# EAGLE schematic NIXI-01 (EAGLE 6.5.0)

## Sheet 1 of 5: Anzeige 1+2
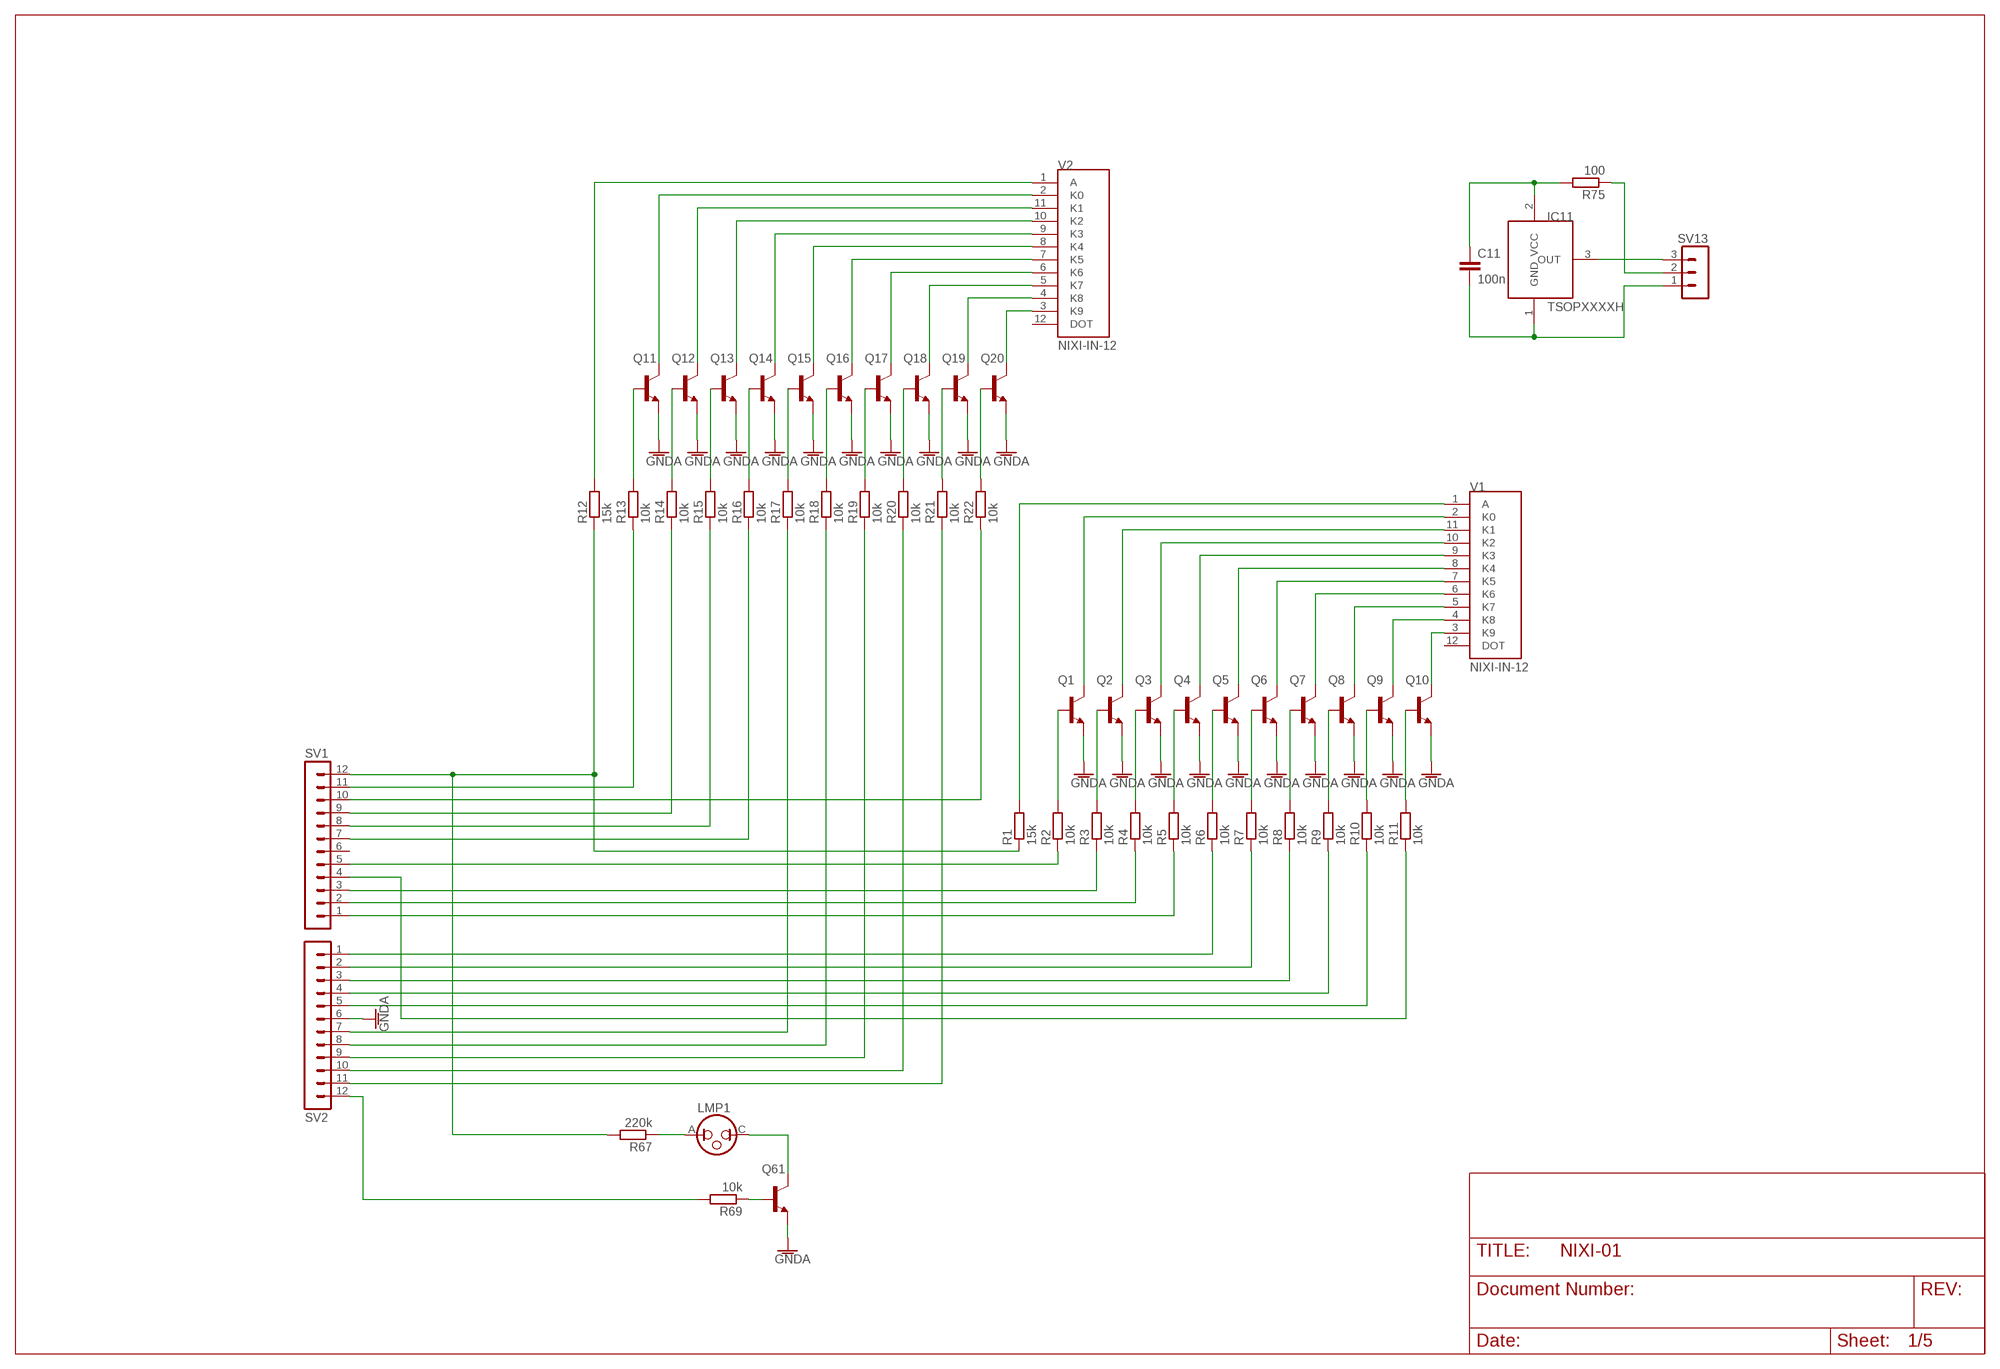
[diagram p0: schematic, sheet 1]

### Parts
C11  100n  C-EUC0603  [C0603]
IC11  TSOPXXXXH  [TSOPXXXX_H]
LMP1  NEON1  [NEONLAMP_6X28]
Q1  BC846ALT1SMD  [SOT23]
Q2  BC846ALT1SMD  [SOT23]
Q3  BC846ALT1SMD  [SOT23]
Q4  BC846ALT1SMD  [SOT23]
Q5  BC846ALT1SMD  [SOT23]
Q6  BC846ALT1SMD  [SOT23]
Q7  BC846ALT1SMD  [SOT23]
Q8  BC846ALT1SMD  [SOT23]
Q9  BC846ALT1SMD  [SOT23]
Q10  BC846ALT1SMD  [SOT23]
Q11  BC846ALT1SMD  [SOT23]
Q12  BC846ALT1SMD  [SOT23]
Q13  BC846ALT1SMD  [SOT23]
Q14  BC846ALT1SMD  [SOT23]
Q15  BC846ALT1SMD  [SOT23]
Q16  BC846ALT1SMD  [SOT23]
Q17  BC846ALT1SMD  [SOT23]
Q18  BC846ALT1SMD  [SOT23]
Q19  BC846ALT1SMD  [SOT23]
Q20  BC846ALT1SMD  [SOT23]
Q61  BC846ALT1SMD  [SOT23]
R1  15k  R-EU_R1206  [R1206]
R2  10k  R-EU_R0603  [R0603]
R3  10k  R-EU_R0603  [R0603]
R4  10k  R-EU_R0603  [R0603]
R5  10k  R-EU_R0603  [R0603]
R6  10k  R-EU_R0603  [R0603]
R7  10k  R-EU_R0603  [R0603]
R8  10k  R-EU_R0603  [R0603]
R9  10k  R-EU_R0603  [R0603]
R10  10k  R-EU_R0603  [R0603]
R11  10k  R-EU_R0603  [R0603]
R12  15k  R-EU_R1206  [R1206]
R13  10k  R-EU_R0603  [R0603]
R14  10k  R-EU_R0603  [R0603]
R15  10k  R-EU_R0603  [R0603]
R16  10k  R-EU_R0603  [R0603]
R17  10k  R-EU_R0603  [R0603]
R18  10k  R-EU_R0603  [R0603]
R19  10k  R-EU_R0603  [R0603]
R20  10k  R-EU_R0603  [R0603]
R21  10k  R-EU_R0603  [R0603]
R22  10k  R-EU_R0603  [R0603]
R67  220k  R-EU_R1206  [R1206]
R69  10k  R-EU_R0603  [R0603]
R75  100  R-EU_R0603  [R0603]
SV1  MA12-1  [MA12-1]
SV2  MA12-1  [MA12-1]
SV13  MA03-1  [MA03-1]
V1  NIXI-IN-12  [NIXI_IN-12]
V2  NIXI-IN-12  [NIXI_IN-12]

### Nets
GNDA: Q1.2(E) Q2.2(E) Q3.2(E) Q4.2(E) Q5.2(E) Q6.2(E) Q7.2(E) Q8.2(E) Q9.2(E) Q10.2(E) Q11.2(E) Q12.2(E) Q13.2(E) Q14.2(E) Q15.2(E) Q16.2(E) Q17.2(E) Q18.2(E) Q19.2(E) Q20.2(E) Q61.2(E) SV2.6 ; also sheet 2,3
N$1: R1.2 V1.1(A)
N$2: Q1.3(C) V1.2(K0)
N$3: Q2.3(C) V1.11(K1)
N$4: Q3.3(C) V1.10(K2)
N$5: Q4.3(C) V1.9(K3)
N$6: Q5.3(C) V1.8(K4)
N$7: Q6.3(C) V1.7(K5)
N$8: Q7.3(C) V1.6(K6)
N$9: Q8.3(C) V1.5(K7)
N$10: Q9.3(C) V1.4(K8)
N$11: Q10.3(C) V1.3(K9)
N$12: Q2.1(B) R3.2
N$13: Q3.1(B) R4.2
N$14: Q4.1(B) R5.2
N$15: Q5.1(B) R6.2
N$16: Q6.1(B) R7.2
N$17: Q7.1(B) R8.2
N$18: Q8.1(B) R9.2
N$19: Q9.1(B) R10.2
N$20: Q10.1(B) R11.2
N$21: Q1.1(B) R2.2
N$22: R5.1 SV1.1
N$23: R4.1 SV1.2
N$24: R3.1 SV1.3
N$25: R11.1 SV1.4
N$26: R2.1 SV1.5
N$28: R6.1 SV2.1
N$29: R7.1 SV2.2
N$30: R8.1 SV2.3
N$31: R9.1 SV2.4
N$32: R10.1 SV2.5
N$33: R12.2 V2.1(A)
N$34: Q11.3(C) V2.2(K0)
N$35: Q12.3(C) V2.11(K1)
N$36: Q13.3(C) V2.10(K2)
N$37: Q14.3(C) V2.9(K3)
N$38: Q15.3(C) V2.8(K4)
N$39: Q16.3(C) V2.7(K5)
N$40: Q17.3(C) V2.6(K6)
N$41: Q18.3(C) V2.5(K7)
N$42: Q19.3(C) V2.4(K8)
N$43: Q20.3(C) V2.3(K9)
N$44: Q12.1(B) R14.2
N$45: Q13.1(B) R15.2
N$46: Q14.1(B) R16.2
N$47: Q15.1(B) R17.2
N$48: Q16.1(B) R18.2
N$49: Q17.1(B) R19.2
N$50: Q18.1(B) R20.2
N$51: Q19.1(B) R21.2
N$52: Q20.1(B) R22.2
N$53: Q11.1(B) R13.2
N$54: R16.1 SV1.7
N$55: R15.1 SV1.8
N$56: R14.1 SV1.9
N$57: R22.1 SV1.10
N$58: R13.1 SV1.11
N$59: R1.1 R12.1 R67.2 SV1.12
N$60: R17.1 SV2.7
N$61: R18.1 SV2.8
N$62: R19.1 SV2.9
N$63: R20.1 SV2.10
N$64: R21.1 SV2.11
N$194: LMP1.C Q61.3(C)
N$195: LMP1.A R67.1
N$196: Q61.1(B) R69.1
N$197: R69.2 SV2.12
N$202: C11.2 IC11.1(GND) SV13.1
N$226: C11.1 IC11.2(VCC) R75.2
N$227: IC11.3(OUT) SV13.3
N$252: R75.1 SV13.2
Unconnected: SV1.6 V1.12(DOT) V2.12(DOT)

## Sheet 2 of 5: Anzeige 3+4
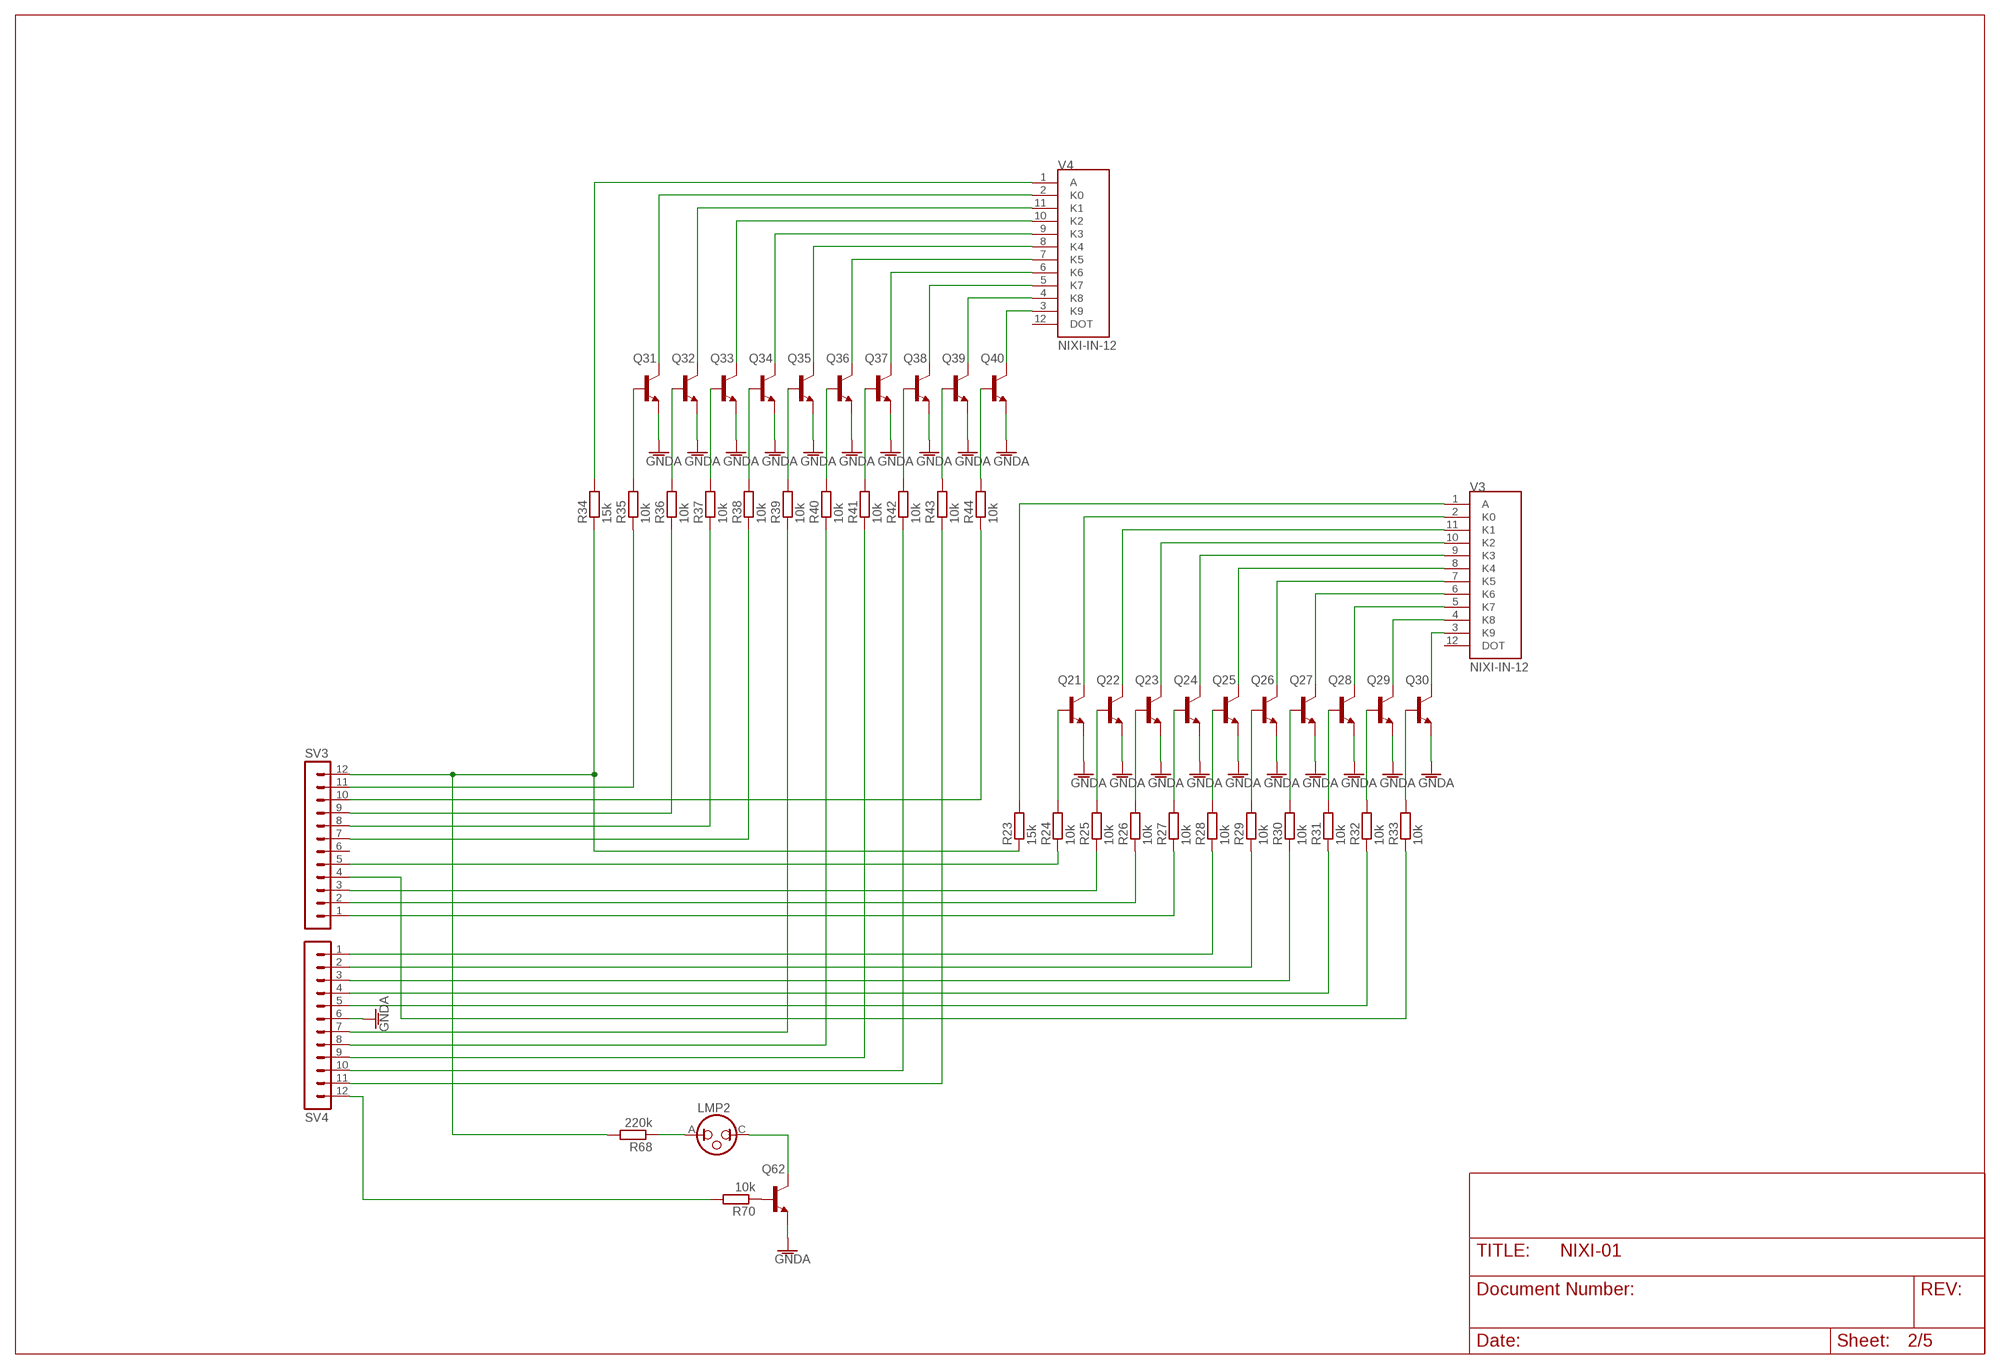
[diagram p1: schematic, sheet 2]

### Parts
LMP2  NEON1  [NEONLAMP_6X28]
Q21  BC846ALT1SMD  [SOT23]
Q22  BC846ALT1SMD  [SOT23]
Q23  BC846ALT1SMD  [SOT23]
Q24  BC846ALT1SMD  [SOT23]
Q25  BC846ALT1SMD  [SOT23]
Q26  BC846ALT1SMD  [SOT23]
Q27  BC846ALT1SMD  [SOT23]
Q28  BC846ALT1SMD  [SOT23]
Q29  BC846ALT1SMD  [SOT23]
Q30  BC846ALT1SMD  [SOT23]
Q31  BC846ALT1SMD  [SOT23]
Q32  BC846ALT1SMD  [SOT23]
Q33  BC846ALT1SMD  [SOT23]
Q34  BC846ALT1SMD  [SOT23]
Q35  BC846ALT1SMD  [SOT23]
Q36  BC846ALT1SMD  [SOT23]
Q37  BC846ALT1SMD  [SOT23]
Q38  BC846ALT1SMD  [SOT23]
Q39  BC846ALT1SMD  [SOT23]
Q40  BC846ALT1SMD  [SOT23]
Q62  BC846ALT1SMD  [SOT23]
R23  15k  R-EU_R1206  [R1206]
R24  10k  R-EU_R0603  [R0603]
R25  10k  R-EU_R0603  [R0603]
R26  10k  R-EU_R0603  [R0603]
R27  10k  R-EU_R0603  [R0603]
R28  10k  R-EU_R0603  [R0603]
R29  10k  R-EU_R0603  [R0603]
R30  10k  R-EU_R0603  [R0603]
R31  10k  R-EU_R0603  [R0603]
R32  10k  R-EU_R0603  [R0603]
R33  10k  R-EU_R0603  [R0603]
R34  15k  R-EU_R1206  [R1206]
R35  10k  R-EU_R0603  [R0603]
R36  10k  R-EU_R0603  [R0603]
R37  10k  R-EU_R0603  [R0603]
R38  10k  R-EU_R0603  [R0603]
R39  10k  R-EU_R0603  [R0603]
R40  10k  R-EU_R0603  [R0603]
R41  10k  R-EU_R0603  [R0603]
R42  10k  R-EU_R0603  [R0603]
R43  10k  R-EU_R0603  [R0603]
R44  10k  R-EU_R0603  [R0603]
R68  220k  R-EU_R1206  [R1206]
R70  10k  R-EU_R0603  [R0603]
SV3  MA12-1  [MA12-1]
SV4  MA12-1  [MA12-1]
V3  NIXI-IN-12  [NIXI_IN-12]
V4  NIXI-IN-12  [NIXI_IN-12]

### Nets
GNDA: Q21.2(E) Q22.2(E) Q23.2(E) Q24.2(E) Q25.2(E) Q26.2(E) Q27.2(E) Q28.2(E) Q29.2(E) Q30.2(E) Q31.2(E) Q32.2(E) Q33.2(E) Q34.2(E) Q35.2(E) Q36.2(E) Q37.2(E) Q38.2(E) Q39.2(E) Q40.2(E) Q62.2(E) SV4.6 ; also sheet 1,3
N$65: R23.2 V3.1(A)
N$66: Q21.3(C) V3.2(K0)
N$67: Q22.3(C) V3.11(K1)
N$68: Q23.3(C) V3.10(K2)
N$69: Q24.3(C) V3.9(K3)
N$70: Q25.3(C) V3.8(K4)
N$71: Q26.3(C) V3.7(K5)
N$72: Q27.3(C) V3.6(K6)
N$73: Q28.3(C) V3.5(K7)
N$74: Q29.3(C) V3.4(K8)
N$75: Q30.3(C) V3.3(K9)
N$76: Q22.1(B) R25.2
N$77: Q23.1(B) R26.2
N$78: Q24.1(B) R27.2
N$79: Q25.1(B) R28.2
N$80: Q26.1(B) R29.2
N$81: Q27.1(B) R30.2
N$82: Q28.1(B) R31.2
N$83: Q29.1(B) R32.2
N$84: Q30.1(B) R33.2
N$85: Q21.1(B) R24.2
N$86: R27.1 SV3.1
N$87: R26.1 SV3.2
N$88: R25.1 SV3.3
N$89: R33.1 SV3.4
N$90: R24.1 SV3.5
N$92: R28.1 SV4.1
N$93: R29.1 SV4.2
N$94: R30.1 SV4.3
N$95: R31.1 SV4.4
N$96: R32.1 SV4.5
N$97: R34.2 V4.1(A)
N$98: Q31.3(C) V4.2(K0)
N$99: Q32.3(C) V4.11(K1)
N$100: Q33.3(C) V4.10(K2)
N$101: Q34.3(C) V4.9(K3)
N$102: Q35.3(C) V4.8(K4)
N$103: Q36.3(C) V4.7(K5)
N$104: Q37.3(C) V4.6(K6)
N$105: Q38.3(C) V4.5(K7)
N$106: Q39.3(C) V4.4(K8)
N$107: Q40.3(C) V4.3(K9)
N$108: Q32.1(B) R36.2
N$109: Q33.1(B) R37.2
N$110: Q34.1(B) R38.2
N$111: Q35.1(B) R39.2
N$112: Q36.1(B) R40.2
N$113: Q37.1(B) R41.2
N$114: Q38.1(B) R42.2
N$115: Q39.1(B) R43.2
N$116: Q40.1(B) R44.2
N$117: Q31.1(B) R35.2
N$118: R38.1 SV3.7
N$119: R37.1 SV3.8
N$120: R36.1 SV3.9
N$121: R44.1 SV3.10
N$122: R35.1 SV3.11
N$124: R39.1 SV4.7
N$125: R40.1 SV4.8
N$126: R41.1 SV4.9
N$127: R42.1 SV4.10
N$128: R43.1 SV4.11
N$193: R23.1 R34.1 R68.2 SV3.12
N$198: LMP2.A R68.1
N$199: LMP2.C Q62.3(C)
N$200: Q62.1(B) R70.1
N$201: R70.2 SV4.12
Unconnected: SV3.6 V3.12(DOT) V4.12(DOT)

## Sheet 3 of 5: Anzeige 5+6
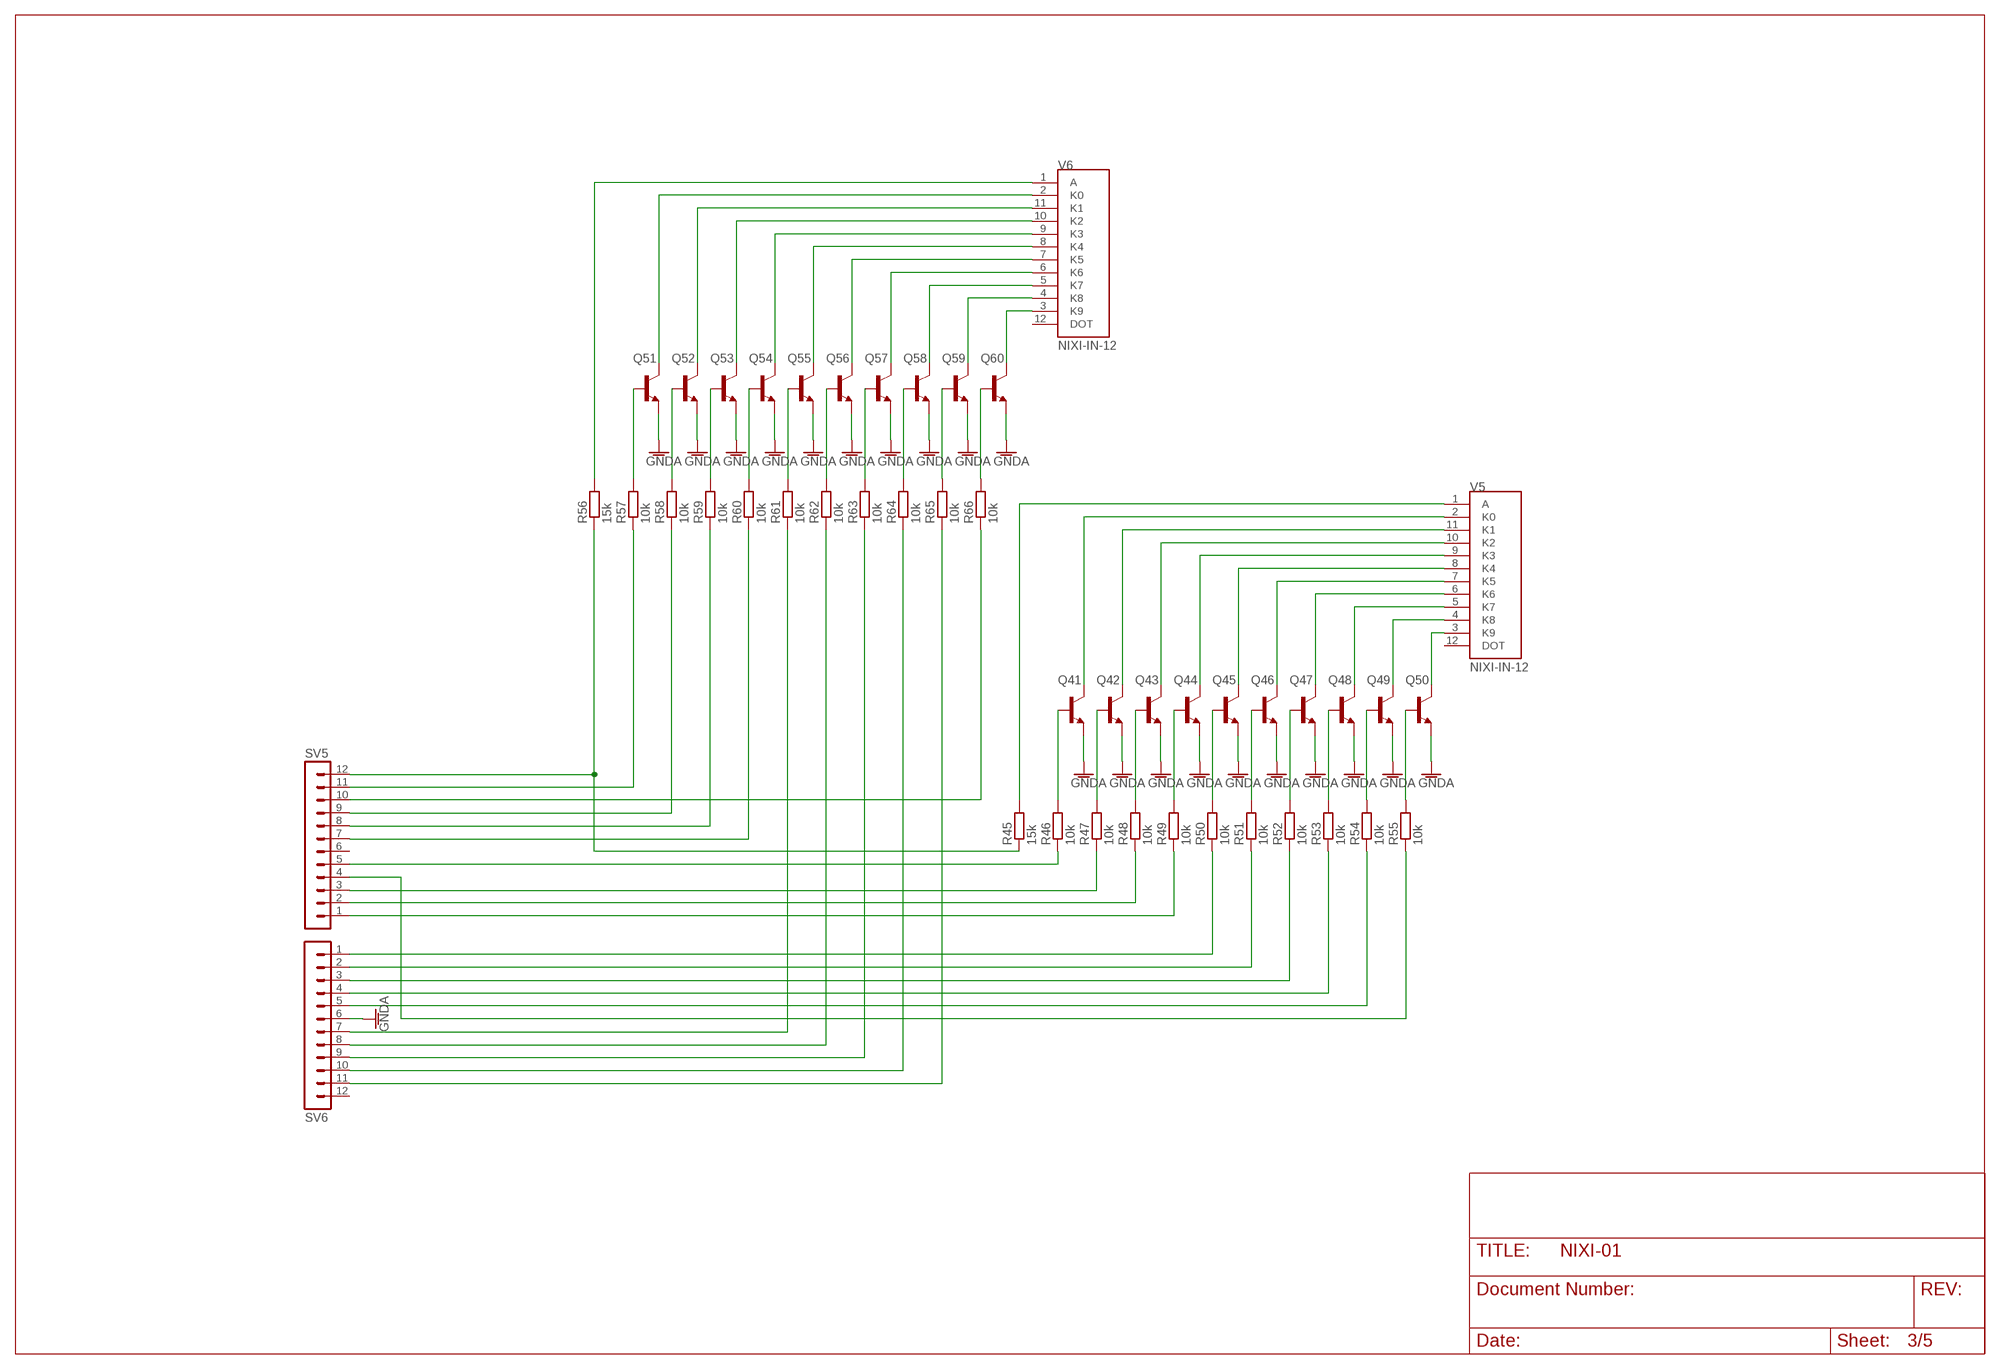
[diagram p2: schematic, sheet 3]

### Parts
Q41  BC846ALT1SMD  [SOT23]
Q42  BC846ALT1SMD  [SOT23]
Q43  BC846ALT1SMD  [SOT23]
Q44  BC846ALT1SMD  [SOT23]
Q45  BC846ALT1SMD  [SOT23]
Q46  BC846ALT1SMD  [SOT23]
Q47  BC846ALT1SMD  [SOT23]
Q48  BC846ALT1SMD  [SOT23]
Q49  BC846ALT1SMD  [SOT23]
Q50  BC846ALT1SMD  [SOT23]
Q51  BC846ALT1SMD  [SOT23]
Q52  BC846ALT1SMD  [SOT23]
Q53  BC846ALT1SMD  [SOT23]
Q54  BC846ALT1SMD  [SOT23]
Q55  BC846ALT1SMD  [SOT23]
Q56  BC846ALT1SMD  [SOT23]
Q57  BC846ALT1SMD  [SOT23]
Q58  BC846ALT1SMD  [SOT23]
Q59  BC846ALT1SMD  [SOT23]
Q60  BC846ALT1SMD  [SOT23]
R45  15k  R-EU_R1206  [R1206]
R46  10k  R-EU_R0603  [R0603]
R47  10k  R-EU_R0603  [R0603]
R48  10k  R-EU_R0603  [R0603]
R49  10k  R-EU_R0603  [R0603]
R50  10k  R-EU_R0603  [R0603]
R51  10k  R-EU_R0603  [R0603]
R52  10k  R-EU_R0603  [R0603]
R53  10k  R-EU_R0603  [R0603]
R54  10k  R-EU_R0603  [R0603]
R55  10k  R-EU_R0603  [R0603]
R56  15k  R-EU_R1206  [R1206]
R57  10k  R-EU_R0603  [R0603]
R58  10k  R-EU_R0603  [R0603]
R59  10k  R-EU_R0603  [R0603]
R60  10k  R-EU_R0603  [R0603]
R61  10k  R-EU_R0603  [R0603]
R62  10k  R-EU_R0603  [R0603]
R63  10k  R-EU_R0603  [R0603]
R64  10k  R-EU_R0603  [R0603]
R65  10k  R-EU_R0603  [R0603]
R66  10k  R-EU_R0603  [R0603]
SV5  MA12-1  [MA12-1]
SV6  MA12-1  [MA12-1]
V5  NIXI-IN-12  [NIXI_IN-12]
V6  NIXI-IN-12  [NIXI_IN-12]

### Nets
GNDA: Q41.2(E) Q42.2(E) Q43.2(E) Q44.2(E) Q45.2(E) Q46.2(E) Q47.2(E) Q48.2(E) Q49.2(E) Q50.2(E) Q51.2(E) Q52.2(E) Q53.2(E) Q54.2(E) Q55.2(E) Q56.2(E) Q57.2(E) Q58.2(E) Q59.2(E) Q60.2(E) SV6.6 ; also sheet 1,2
N$129: R45.2 V5.1(A)
N$130: Q41.3(C) V5.2(K0)
N$131: Q42.3(C) V5.11(K1)
N$132: Q43.3(C) V5.10(K2)
N$133: Q44.3(C) V5.9(K3)
N$134: Q45.3(C) V5.8(K4)
N$135: Q46.3(C) V5.7(K5)
N$136: Q47.3(C) V5.6(K6)
N$137: Q48.3(C) V5.5(K7)
N$138: Q49.3(C) V5.4(K8)
N$139: Q50.3(C) V5.3(K9)
N$140: Q42.1(B) R47.2
N$141: Q43.1(B) R48.2
N$142: Q44.1(B) R49.2
N$143: Q45.1(B) R50.2
N$144: Q46.1(B) R51.2
N$145: Q47.1(B) R52.2
N$146: Q48.1(B) R53.2
N$147: Q49.1(B) R54.2
N$148: Q50.1(B) R55.2
N$149: Q41.1(B) R46.2
N$150: R49.1 SV5.1
N$151: R48.1 SV5.2
N$152: R47.1 SV5.3
N$153: R55.1 SV5.4
N$154: R46.1 SV5.5
N$156: R50.1 SV6.1
N$157: R51.1 SV6.2
N$158: R52.1 SV6.3
N$159: R53.1 SV6.4
N$160: R54.1 SV6.5
N$161: R56.2 V6.1(A)
N$162: Q51.3(C) V6.2(K0)
N$163: Q52.3(C) V6.11(K1)
N$164: Q53.3(C) V6.10(K2)
N$165: Q54.3(C) V6.9(K3)
N$166: Q55.3(C) V6.8(K4)
N$167: Q56.3(C) V6.7(K5)
N$168: Q57.3(C) V6.6(K6)
N$169: Q58.3(C) V6.5(K7)
N$170: Q59.3(C) V6.4(K8)
N$171: Q60.3(C) V6.3(K9)
N$172: Q52.1(B) R58.2
N$173: Q53.1(B) R59.2
N$174: Q54.1(B) R60.2
N$175: Q55.1(B) R61.2
N$176: Q56.1(B) R62.2
N$177: Q57.1(B) R63.2
N$178: Q58.1(B) R64.2
N$179: Q59.1(B) R65.2
N$180: Q60.1(B) R66.2
N$181: Q51.1(B) R57.2
N$182: R60.1 SV5.7
N$183: R59.1 SV5.8
N$184: R58.1 SV5.9
N$185: R66.1 SV5.10
N$186: R57.1 SV5.11
N$187: R45.1 R56.1 SV5.12
N$188: R61.1 SV6.7
N$189: R62.1 SV6.8
N$190: R63.1 SV6.9
N$191: R64.1 SV6.10
N$192: R65.1 SV6.11
Unconnected: SV5.6 SV6.12 V5.12(DOT) V6.12(DOT)

## Sheet 4 of 5: Schieberegister
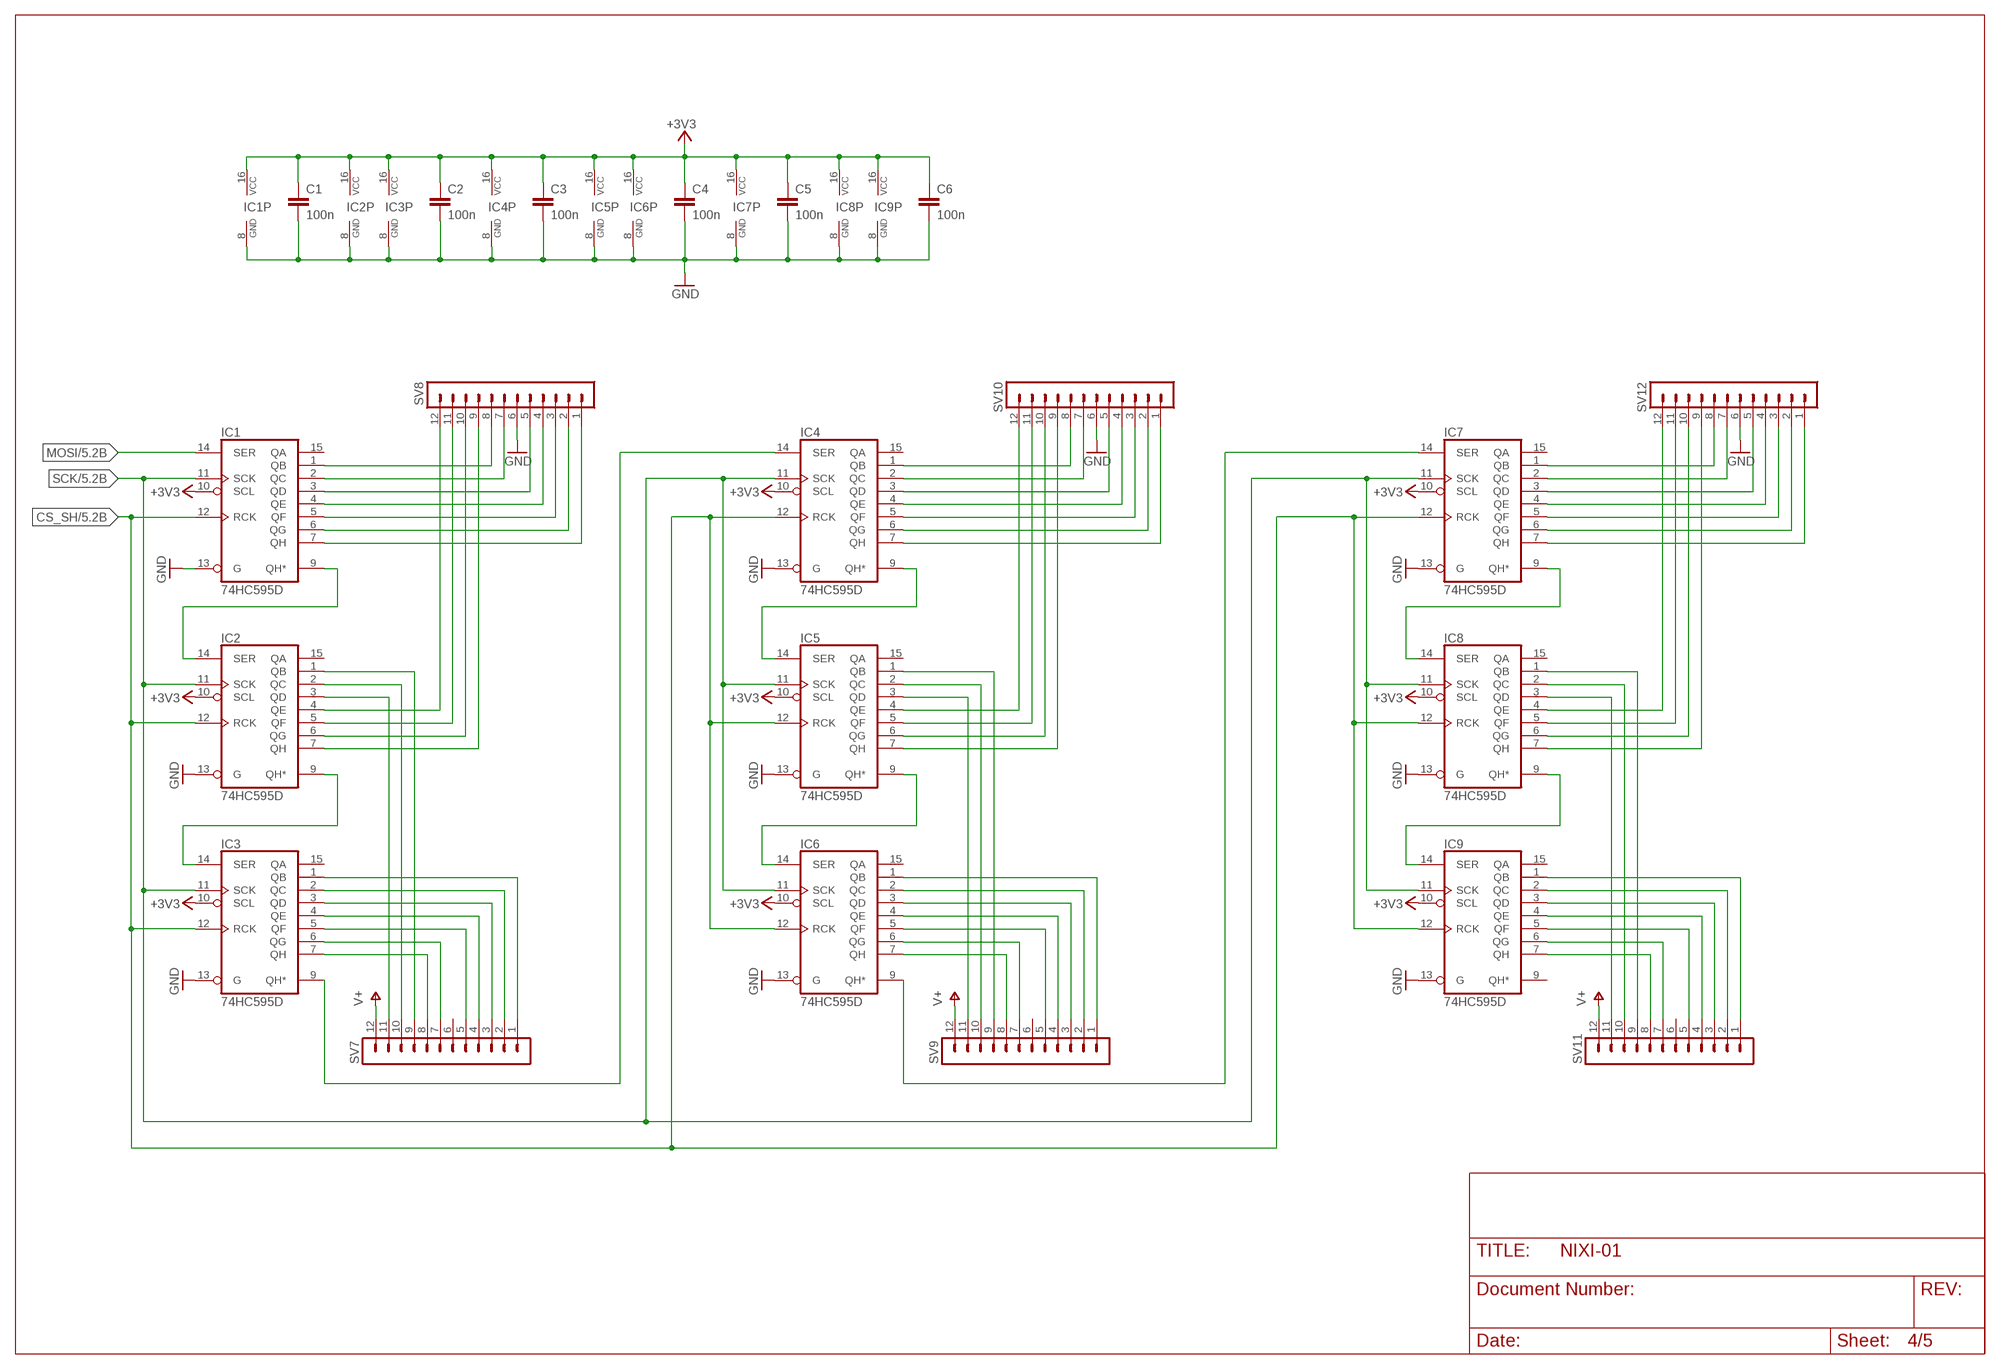
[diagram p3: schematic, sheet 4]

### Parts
C1  100n  C-EUC0603  [C0603]
C2  100n  C-EUC0603  [C0603]
C3  100n  C-EUC0603  [C0603]
C4  100n  C-EUC0603  [C0603]
C5  100n  C-EUC0603  [C0603]
C6  100n  C-EUC0603  [C0603]
IC1  74HC595D  [SO16]
IC2  74HC595D  [SO16]
IC3  74HC595D  [SO16]
IC4  74HC595D  [SO16]
IC5  74HC595D  [SO16]
IC6  74HC595D  [SO16]
IC7  74HC595D  [SO16]
IC8  74HC595D  [SO16]
IC9  74HC595D  [SO16]
SV7  MA12-1  [MA12-1]
SV8  MA12-1  [MA12-1]
SV9  MA12-1  [MA12-1]
SV10  MA12-1  [MA12-1]
SV11  MA12-1  [MA12-1]
SV12  MA12-1  [MA12-1]

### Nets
+3V3: C1.1 C2.1 C3.1 C4.1 C5.1 C6.1 IC1.10(SCL) IC1.16(VCC) IC2.10(SCL) IC2.16(VCC) IC3.10(SCL) IC3.16(VCC) IC4.10(SCL) IC4.16(VCC) IC5.10(SCL) IC5.16(VCC) IC6.10(SCL) IC6.16(VCC) IC7.10(SCL) IC7.16(VCC) IC8.10(SCL) IC8.16(VCC) IC9.10(SCL) IC9.16(VCC) ; also sheet 5
CS_SH: IC1.12(RCK) IC2.12(RCK) IC3.12(RCK) IC4.12(RCK) IC5.12(RCK) IC6.12(RCK) IC7.12(RCK) IC8.12(RCK) IC9.12(RCK) ; also sheet 5
GND: C1.2 C2.2 C3.2 C4.2 C5.2 C6.2 IC1.8(GND) IC1.13(G) IC2.8(GND) IC2.13(G) IC3.8(GND) IC3.13(G) IC4.8(GND) IC4.13(G) IC5.8(GND) IC5.13(G) IC6.8(GND) IC6.13(G) IC7.8(GND) IC7.13(G) IC8.8(GND) IC8.13(G) IC9.8(GND) IC9.13(G) SV8.6 SV10.6 SV12.6 ; also sheet 5
MOSI: IC1.14(SER) ; also sheet 5
N$27: IC1.9(QH*) IC2.14(SER)
N$91: IC2.9(QH*) IC3.14(SER)
N$203: IC1.7(QH) SV8.1
N$204: IC1.6(QG) SV8.2
N$205: IC1.5(QF) SV8.3
N$206: IC1.4(QE) SV8.4
N$207: IC1.3(QD) SV8.5
N$208: IC1.2(QC) SV8.7
N$209: IC1.1(QB) SV8.8
N$210: IC2.7(QH) SV8.9
N$211: IC2.6(QG) SV8.10
N$212: IC2.5(QF) SV8.11
N$213: IC2.4(QE) SV8.12
N$214: IC3.1(QB) SV7.1
N$215: IC3.2(QC) SV7.2
N$216: IC3.3(QD) SV7.3
N$217: IC3.4(QE) SV7.4
N$218: IC3.5(QF) SV7.5
N$219: IC3.6(QG) SV7.7
N$220: IC3.7(QH) SV7.8
N$221: IC2.1(QB) SV7.9
N$222: IC2.2(QC) SV7.10
N$223: IC2.3(QD) SV7.11
N$224: IC4.9(QH*) IC5.14(SER)
N$225: IC5.9(QH*) IC6.14(SER)
N$228: IC3.9(QH*) IC4.14(SER)
N$229: IC4.7(QH) SV10.1
N$230: IC4.6(QG) SV10.2
N$231: IC4.5(QF) SV10.3
N$232: IC4.4(QE) SV10.4
N$233: IC4.3(QD) SV10.5
N$234: IC4.2(QC) SV10.7
N$235: IC4.1(QB) SV10.8
N$236: IC5.7(QH) SV10.9
N$237: IC5.6(QG) SV10.10
N$238: IC5.5(QF) SV10.11
N$239: IC5.4(QE) SV10.12
N$240: IC6.1(QB) SV9.1
N$241: IC6.2(QC) SV9.2
N$242: IC6.3(QD) SV9.3
N$243: IC6.4(QE) SV9.4
N$244: IC6.5(QF) SV9.5
N$245: IC6.6(QG) SV9.7
N$246: IC6.7(QH) SV9.8
N$247: IC5.1(QB) SV9.9
N$248: IC5.2(QC) SV9.10
N$249: IC5.3(QD) SV9.11
N$250: IC7.9(QH*) IC8.14(SER)
N$251: IC8.9(QH*) IC9.14(SER)
N$254: IC6.9(QH*) IC7.14(SER)
N$255: IC7.7(QH) SV12.1
N$256: IC7.6(QG) SV12.2
N$257: IC7.5(QF) SV12.3
N$258: IC7.4(QE) SV12.4
N$259: IC7.3(QD) SV12.5
N$260: IC7.2(QC) SV12.7
N$261: IC7.1(QB) SV12.8
N$262: IC8.7(QH) SV12.9
N$263: IC8.6(QG) SV12.10
N$264: IC8.5(QF) SV12.11
N$265: IC8.4(QE) SV12.12
N$266: IC9.1(QB) SV11.1
N$267: IC9.2(QC) SV11.2
N$268: IC9.3(QD) SV11.3
N$269: IC9.4(QE) SV11.4
N$270: IC9.5(QF) SV11.5
N$271: IC9.6(QG) SV11.7
N$272: IC9.7(QH) SV11.8
N$273: IC8.1(QB) SV11.9
N$274: IC8.2(QC) SV11.10
N$275: IC8.3(QD) SV11.11
SCK: IC1.11(SCK) IC2.11(SCK) IC3.11(SCK) IC4.11(SCK) IC5.11(SCK) IC6.11(SCK) IC7.11(SCK) IC8.11(SCK) IC9.11(SCK) ; also sheet 5
V+: SV7.12 SV9.12 SV11.12 ; also sheet 5
Unconnected: IC1.15(QA) IC2.15(QA) IC3.15(QA) IC4.15(QA) IC5.15(QA) IC6.15(QA) IC7.15(QA) IC8.15(QA) IC9.9(QH*) IC9.15(QA) SV7.6 SV9.6 SV11.6

## Sheet 5 of 5: CPU
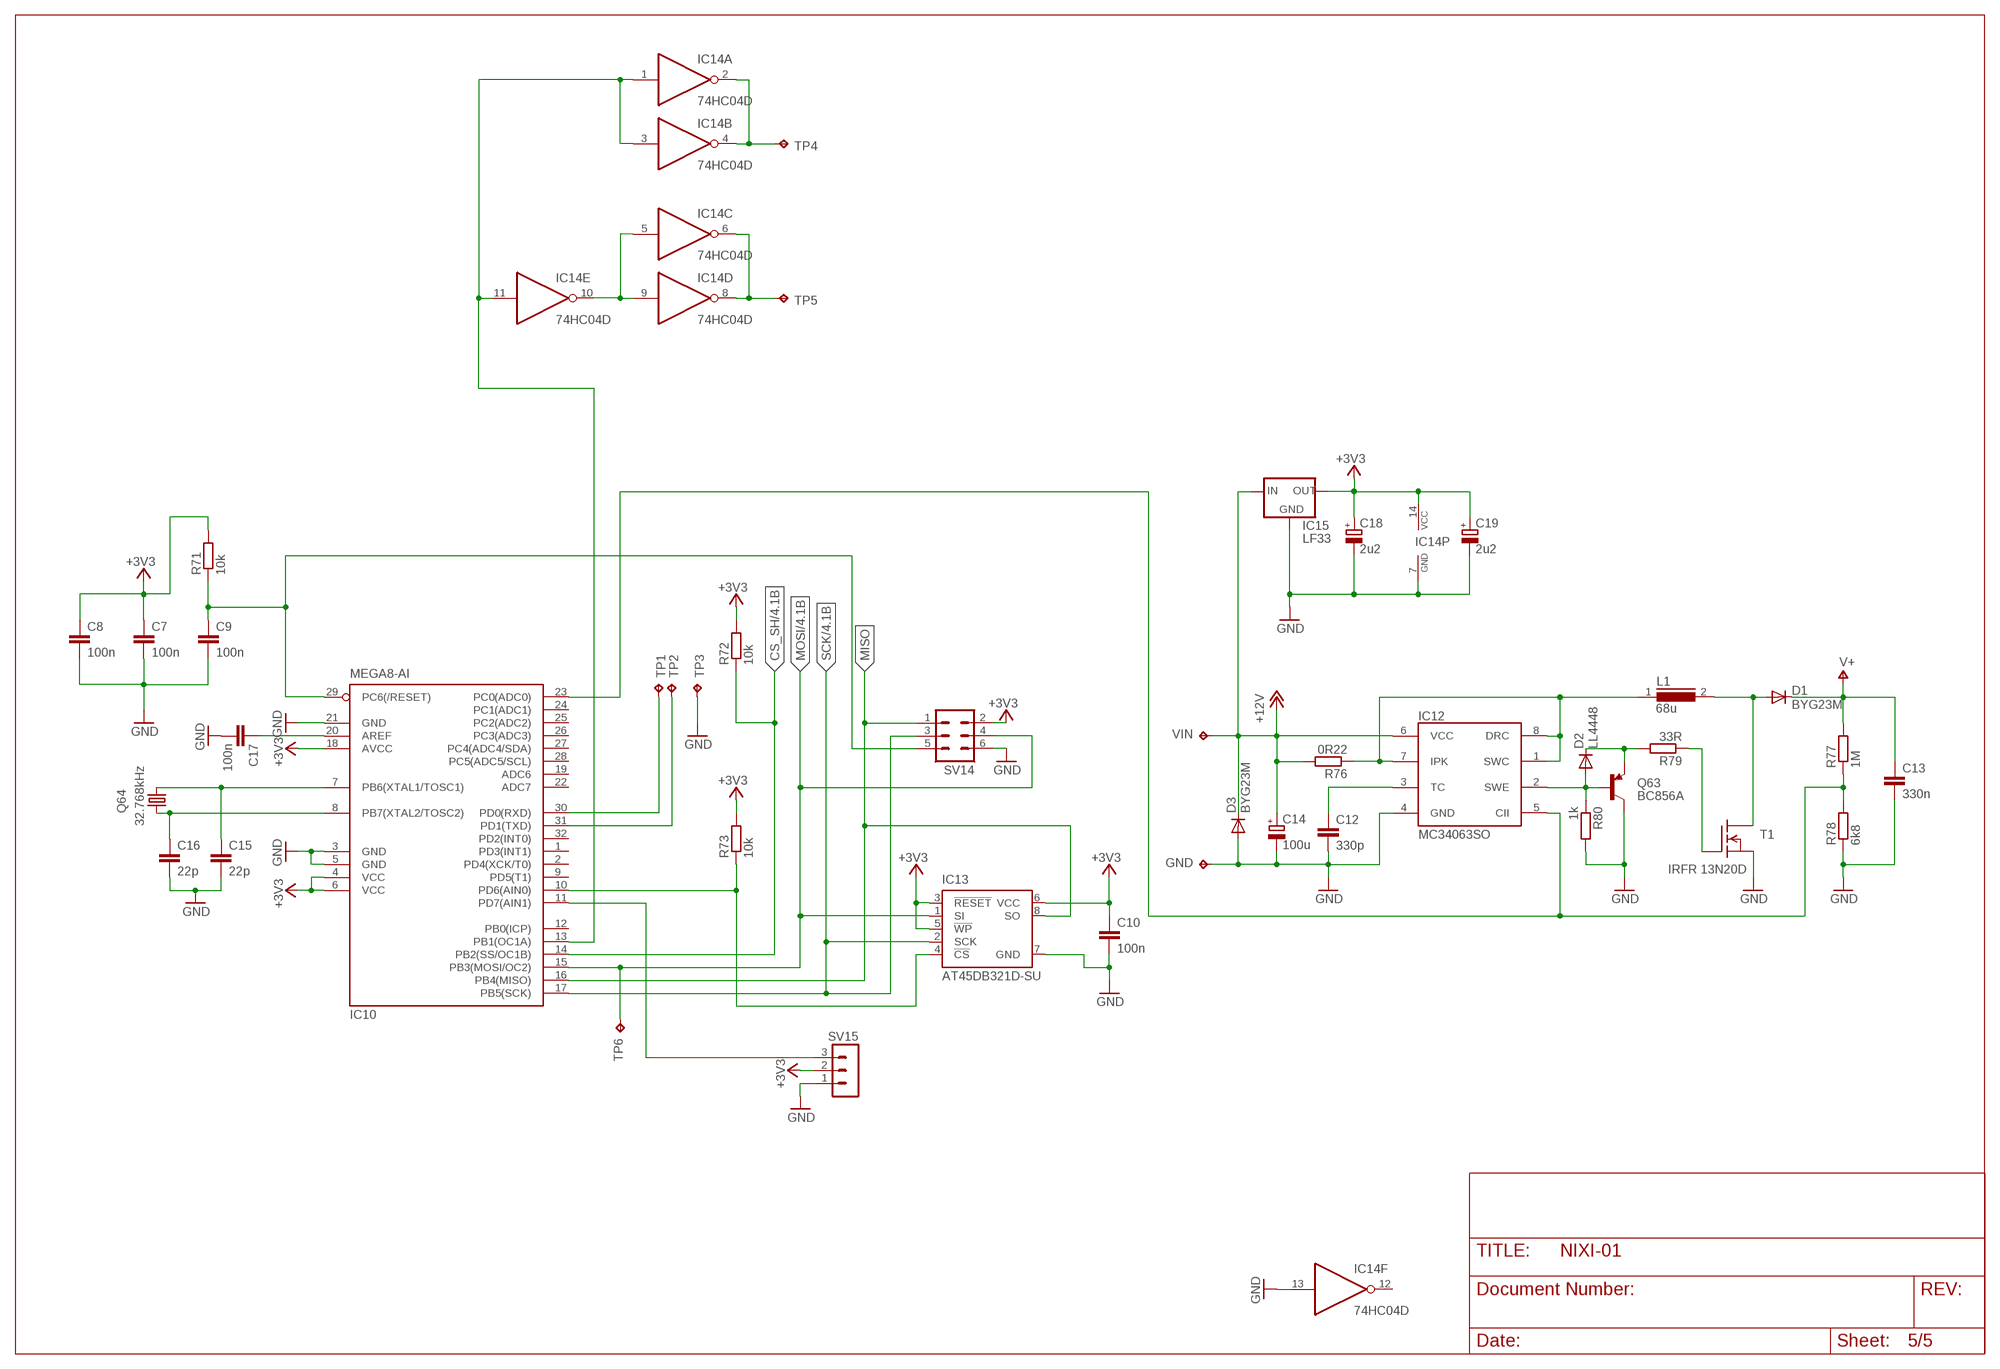
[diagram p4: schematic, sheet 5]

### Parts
C7  100n  C-EUC0603  [C0603]
C8  100n  C-EUC0603  [C0603]
C9  100n  C-EUC0603  [C0603]
C10  100n  C-EUC0603  [C0603]
C12  330p  C-EUC0603  [C0603]
C13  330n  C-EU150-054X183  [C150-054X183]
C14  100u  CPOL-EU153CLV-0810  [153CLV-0810]
C15  22p  C-EUC0603  [C0603]
C16  22p  C-EUC0603  [C0603]
C17  100n  C-EUC0603  [C0603]
C18  2u2  CPOL-EUSMCA  [SMC_A]
C19  2u2  CPOL-EUSMCA  [SMC_A]
D1  BYG23M  DIODE-DO-214AC  [DO-214AC]
D2  LL4448  DIODE-MICROMELF-W  [MICROMELF-W]
D3  BYG23M  DIODE-DO-214AC  [DO-214AC]
GND  TPPAD1-13  [P1-13]
IC10  MEGA8-AI  [TQFP32-08]
IC12  MC34063SO  [SO-08]
IC13  AT45DB321D-SU  AT45DB161D-SU  [8S2]
IC14  74HC04D  [SO14]
IC15  LF33  LF00  [DPACK_1]
L1  68u  DR125  [DR125]
Q63  BC856A  BC856ASMD  [SOT23-BEC]
Q64  32.768kHz  CRYSTALTC38H  [TC38H]
R71  10k  R-EU_R0603  [R0603]
R72  10k  R-EU_R0603  [R0603]
R73  10k  R-EU_R0603  [R0603]
R76  0R22  R-EU_R1206  [R1206]
R77  1M  R-EU_R1206  [R1206]
R78  6k8  R-EU_R0603  [R0603]
R79  33R  R-EU_R0603  [R0603]
R80  1k  R-EU_R0603  [R0603]
SV14  ML6  [ML6]
SV15  MA03-1  [MA03-1]
T1  IRFR 13N20D  BUZ11DPACK  [DPACK_1]
TP1  TPPAD1-13  [P1-13]
TP2  TPPAD1-13  [P1-13]
TP3  TPPAD1-13  [P1-13]
TP4  TPP1-06  [P1-06]
TP5  TPP1-06  [P1-06]
TP6  TPP1-06  [P1-06]
VIN  TPPAD1-13  [P1-13]

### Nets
+3V3: C7.1 C8.1 C10.1 C18.+ C19.+ IC10.4(VCC) IC10.6(VCC) IC10.18(AVCC) IC13.3(!RESET) IC13.5(!WP) IC13.6(VCC) IC14.14(P:VCC) IC15.2(OUT) R71.2 R72.2 R73.2 SV14.2 SV15.2 ; also sheet 4
+12V: C14.+ D3.C IC12.6(VCC) IC15.1(IN) R76.2 VIN.TP
CS_SH: IC10.14(PB2(SS/OC1B)) R72.1 ; also sheet 4
GND: C7.2 C8.2 C9.2 C10.2 C12.2 C13.2 C14.- C15.2 C16.2 C17.2 C18.- C19.- D3.A GND.TP IC10.3(GND) IC10.5(GND) IC10.21(GND) IC12.4(GND) IC13.7(GND) IC14.7(P:GND) IC14.13(F:I) IC15.3(GND) Q63.C R78.1 R80.2 SV14.6 SV15.1 T1.2(S) TP3.TP ; also sheet 4
MISO: IC10.16(PB4(MISO)) IC13.8(SO) SV14.1
MOSI: IC10.15(PB3(MOSI/OC2)) IC13.1(SI) SV14.4 TP6.TP ; also sheet 4
N$123: C17.1 IC10.20(AREF)
N$155: C9.1 IC10.29(PC6(/RESET)) R71.1 SV14.5
N$253: IC12.1(SWC) IC12.7(IPK) IC12.8(DRC) L1.1 R76.1
N$276: D2.A IC12.2(SWE) Q63.B R80.1
N$277: C12.1 IC12.3(TC)
N$278: D1.A L1.2 T1.3(D)
N$279: IC10.23(PC0(ADC0)) IC12.5(CII) R77.1 R78.2
N$280: D2.C Q63.E R79.2
N$281: R79.1 T1.1(G)
N$282: IC10.11(PD7(AIN1)) SV15.3
N$283: IC10.30(PD0(RXD)) TP1.TP
N$284: IC10.31(PD1(TXD)) TP2.TP
N$285: IC14.5(C:I) IC14.9(D:I) IC14.10(E:O)
N$287: IC10.10(PD6(AIN0)) IC13.4(!CS) R73.1
N$288: IC14.2(A:O) IC14.4(B:O) TP4.TP
N$289: C15.1 IC10.7(PB6(XTAL1/TOSC1)) Q64.2
N$290: C16.1 IC10.8(PB7(XTAL2/TOSC2)) Q64.1
N$291: IC14.6(C:O) IC14.8(D:O) TP5.TP
N$292: IC10.13(PB1(OC1A)) IC14.1(A:I) IC14.3(B:I) IC14.11(E:I)
SCK: IC10.17(PB5(SCK)) IC13.2(SCK) SV14.3 ; also sheet 4
V+: C13.1 D1.C R77.2 ; also sheet 4
Unconnected: IC10.1(PD3(INT1)) IC10.2(PD4(XCK/T0)) IC10.9(PD5(T1)) IC10.12(PB0(ICP)) IC10.19(ADC6) IC10.22(ADC7) IC10.24(PC1(ADC1)) IC10.25(PC2(ADC2)) IC10.26(PC3(ADC3)) IC10.27(PC4(ADC4/SDA)) IC10.28(PC5(ADC5/SCL)) IC10.32(PD2(INT0)) IC14.12(F:O)

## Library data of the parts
C1-C13 C15-C17 = rcl:C-EU: CAPACITOR, European symbol
C14 C18 C19 = rcl:CPOL-EU: POLARIZED CAPACITOR, European symbol
D1-D3 = diode:DIODE-: DIODE
GND TP1-TP6 VIN = testpad:TP: Test pad
IC1-IC9 = 74xx-eu:74*595: 8-bit SHIFT REGISTER, output latch
IC10 = atmel:MEGA8: MICROCONTROLLER 8 Kbytes FLASH, 1 kbytes SRAM, 512 bytes EEPROM, USART, 6-channel 10 bit ADC, 2-channel 8 bit ADC Pin compatible with Atmega48, ATMega88, ATMega168 Source: avr.lbr; MPN: ATMEGA8-16AU; OC_FARNELL: 9171371; OC_NEWARK: 73M8863
IC11 = Brunner:TSOPXXXX
IC12 = Brunner:MC34063
IC13 = atmel:AT45DB161D: 16-megabit 2.5V or 2.7V DataFlash Source: http://www.atmel.com/dyn/resources/prod_documents/doc3500.pdf; MF: ATMEL; MPN: AT45DB161D-SU; OC_FARNELL: 1455040
IC14 = 74xx-eu:74*04: Hex INVERTER
IC15 = Brunner:LF00
L1 = inductors:DR125: High Power Density, High Efficiency, Shielded Inductors
LMP1 LMP2 = Brunner:NEON: Neon LAMP
Q1-Q62 = transistor-npn:BC846*: NPN Transistor
Q63 = transistor-pnp:BC856*: PNP Transistror
Q64 = crystal:CRYSTAL: CRYSTAL; OC_FARNELL: unknown; OC_NEWARK: unknown
R1-R73 R75-R80 = rcl:R-EU_: RESISTOR, European symbol
SV1-SV12 = con-lstb:MA12-1: PIN HEADER; OC_FARNELL: unknown; OC_NEWARK: unknown
SV13 SV15 = con-lstb:MA03-1: PIN HEADER; OC_FARNELL: unknown; OC_NEWARK: unknown
SV14 = con-harting-ml:ML6: HARTING; OC_FARNELL: unknown; OC_NEWARK: unknown
T1 = Brunner:BUZ11: N-Channel Enhancement MOSFET 50V; 30A; 0,040Ohm
V1-V6 = Brunner:NIXI-IN-12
